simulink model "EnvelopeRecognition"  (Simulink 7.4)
settings: Solver=FixedStepDiscrete  StartTime=0.0  StopTime=10.0  RelTol=1e-3
undefined symbols (not defined in the file or in its folder): Rec, SDTV, uint
libraries: viptextngfix x3, vipconversions x3, vipsnks x2, vipmorphops x1, vipsrcs x1, dspmtrx3 x1

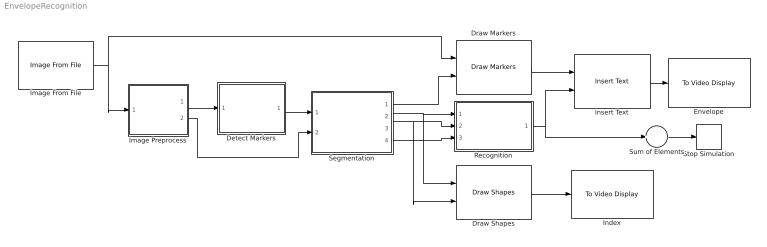
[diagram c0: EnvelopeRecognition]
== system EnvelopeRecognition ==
  Detect Markers : Subsystem
  Draw Markers : viptextngfix/Draw Markers  DialogController=vipDDGCreate  DialogControllerArgs=DataTag0  shape=X-mark  size=10  fill=on  fillClrSource=Specify via dialog  display=User-specified value  intensity=200  color=[200 255 100]  opacity=0.6  viewport=Entire image  antialiasing=off  inType=Obsolete  imagePorts=One multidimensional signal  prodOutputMode=Binary point scaling  prodOutputWordLength=32  prodOutputFracLength=14  memoryMode=Specify word length  memoryWordLength=16  memoryFracLength=15  roundingMode=Floor  overflowMode=off
  Draw Shapes : viptextngfix/Draw Shapes  DialogController=vipDDGCreate  DialogControllerArgs=DataTag1  shape=Rectangles  fill=off  fillClrSource=Specify via dialog  display=White  intensity=200  color=[0 255 0]'*ones(1, 7)  opacity=0.6  viewport=Entire image  antialiasing=off  inType=Obsolete  imagePorts=One multidimensional signal  prodOutputMode=Binary point scaling  prodOutputWordLength=32  prodOutputFracLength=14  memoryMode=Specify word length  memoryWordLength=16  memoryFracLength=15  roundingMode=Floor  overflowMode=off
  Envelope : vipsnks/To Video Display  DialogControllerArgs=DataTag2  inputType=Obsolete  imagePorts=One multidimensional signal  OutputDevice=On-screen video monitor  fullScreen=off  videoWindowX=48  videoWindowY=189  saveWindowSize=off  videoWindowWidth=1152  videoWindowHeight=757  dataOrg=Column-major  openAtMdlStart=on  isWindowOpen=off
  Image From File : vipsrcs/Image From File  Tag=vipblks_nd  DialogController=vipDDGCreate  DialogControllerArgs=DataTag3  SystemSampleTime=-1  FileName=E:\KPI\C_V_S\RGR\RELEASE\Images\DSC00377.JPG  imagePorts=One multidimensional signal  Ts=inf  ImageDataType=Inherit from input image  Signed=on  WordLength=16  sdImageDataType=uint(8)  FractionLengthMode=User-defined  FractionLength=15  OutPortLabels=R|G|B
  Image Preprocess : Subsystem
  Index : vipsnks/To Video Display  DialogControllerArgs=DataTag5  inputType=Obsolete  imagePorts=One multidimensional signal  OutputDevice=On-screen video monitor  fullScreen=off  videoWindowX=179  videoWindowY=214  saveWindowSize=off  videoWindowWidth=217  videoWindowHeight=65  dataOrg=Column-major  openAtMdlStart=on  isWindowOpen=off
  Insert Text : viptextngfix/Insert Text  DialogController=vipDDGCreate  DialogControllerArgs=DataTag6  inputType=Obsolete  theText='%s'  fontFace=Arial  dummyVar1=0  blockFontSize=48  antiAliased=on  getTextLocFrom=Specify via dialog  textLoc=[0 0]  getTextColorFrom=Specify via dialog  textColor=[0 255 0]  getTextIntensityFrom=Specify via dialog  textIntensity=0  getTextOpacityFrom=Specify via dialog  textOpacity=1.0  dummyVar2=0  dummyVar3=0  dummyVar4=0  imagePorts=One multidimensional signal  isInputTransposed=off
  Recognition : Subsystem
  Segmentation : Subsystem
  Stop Simulation : Stop
  Sum of Elements : Sum  Inputs=+  OutDataTypeMode=double  OutDataType=fixdt(1, 16)  OutScaling=2^-10  OutDataTypeStr=double
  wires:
  Image From File/1 -> Draw Markers/1, Image Preprocess/1(Image)
  Image Preprocess/1(BW) -> Detect Markers/1(BWin)
  Detect Markers/1(STATS) -> Segmentation/1(STATS)
  Segmentation/1(Pts) -> Draw Markers/2
  Image Preprocess/2(Gray) -> Segmentation/2(Image)
  Draw Shapes/1 -> Index/1
  Segmentation/2(IndexImage) -> Draw Shapes/1, Recognition/1(IndexImage)
  Segmentation/3(Rects) -> Draw Shapes/2, Recognition/2(Rects)
  Segmentation/4(Thresh) -> Recognition/3(Thresh)
  Draw Markers/1 -> Insert Text/1
  Insert Text/1 -> Envelope/1
  Recognition/1(Index) -> Insert Text/2, Sum of Elements/1
  Sum of Elements/1 -> Stop Simulation/1

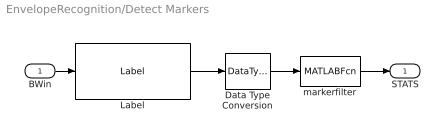
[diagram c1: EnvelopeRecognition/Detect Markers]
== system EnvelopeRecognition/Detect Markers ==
  BWin : Inport  OutDataType=fixdt(1, 16)  OutScaling=2^0
  Data Type Conversion : DataTypeConversion  OutDataTypeMode=double  OutDataType=fixdt(1, 16)  OutScaling=2^0  OutDataTypeStr=double
  Label : vipmorphops/Label  conn=8  output=Label matrix  outType=Automatic  lastLabel=maximum value of the output data type
  markerfilter : MATLABFcn  MATLABFcn=markerfilter  OutputDimensions=[7, 7]  Output1D=off
  STATS : Outport  OutDataType=fixdt(1, 16)  OutScaling=2^0
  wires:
  BWin/1 -> Label/1
  Label/1 -> Data Type Conversion/1
  markerfilter/1 -> STATS/1
  Data Type Conversion/1 -> markerfilter/1

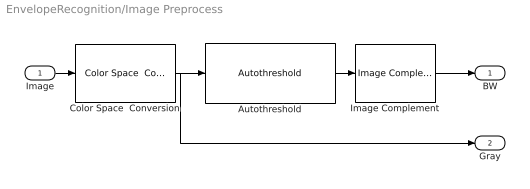
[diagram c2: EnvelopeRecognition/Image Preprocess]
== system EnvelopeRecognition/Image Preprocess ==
  Image : Inport  OutDataType=fixdt(1, 16)  OutScaling=2^0
  Autothreshold : vipconversions/Autothreshold  DialogController=vipDDGCreate  DialogControllerArgs=DataTag4  operator=>  threshOut=off  effMetricOut=off  userDefinedRange=off  umin=0  umax=255  outOfRngOpt=Warn and saturate  scaleThreshold=off  scaleFactor=1  P1Mode=Specify word length  P1WordLength=32  P1FracLength=30  P2Mode=Specify word length  P2WordLength=32  P2FracLength=22  P3Mode=Specify word length  P3WordLength=32  P3FracLength=14  P4Mode=Binary point scaling  P4WordLength=32  P4FracLength=15  Q1Mode=Specify word length  Q1WordLength=32  Q1FracLength=16  EMMode=Specify word length  EMWordLength=16  EMFracLength=14  roundingMode=Floor  overflowMode=off
  Color Space  Conversion : vipconversions/Color Space  Conversion  conversion=Obsolete  conversionActive=R'G'B' to intensity  wp_str=D65  rec=Rec. 601 (SDTV)  sys=1125/60/2:1  imagePorts=One multidimensional signal
  Image Complement : vipconversions/Image Complement
  BW : Outport  OutDataType=fixdt(1, 16)  OutScaling=2^0
  Gray : Outport  Port=2  OutDataType=fixdt(1, 16)  OutScaling=2^0
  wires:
  Image/1 -> Color Space  Conversion/1
  Color Space  Conversion/1 -> Autothreshold/1, Gray/1
  Autothreshold/1 -> Image Complement/1
  Image Complement/1 -> BW/1

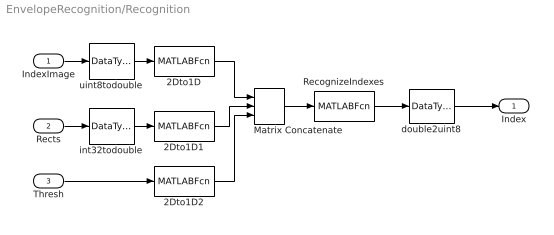
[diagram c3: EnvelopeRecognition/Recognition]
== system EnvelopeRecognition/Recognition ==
  IndexImage : Inport  OutDataType=fixdt(1, 16)  OutScaling=2^0
  Rects : Inport  Port=2  OutDataType=fixdt(1, 16)  OutScaling=2^0
  Thresh : Inport  Port=3  OutDataType=fixdt(1, 16)  OutScaling=2^0
  2Dto1D : MATLABFcn  MATLABFcn=transform2Dto1D
  2Dto1D1 : MATLABFcn  MATLABFcn=transform2Dto1D
  2Dto1D2 : MATLABFcn  MATLABFcn=transform2Dto1D
  Matrix Concatenate : Concatenate  NumInputs=3  Mode=Vector  ConcatenateDimension=2
  RecognizeIndexes : MATLABFcn  MATLABFcn=recognizeindexes  OutputDimensions=[1, 6]  Output1D=off
  double2uint8 : DataTypeConversion  OutDataTypeMode=uint8  OutDataType=fixdt(1, 16)  OutScaling=2^0  OutDataTypeStr=uint8
  int32todouble : DataTypeConversion  OutDataTypeMode=double  OutDataType=fixdt(1, 16)  OutScaling=2^0  OutDataTypeStr=double
  uint8todouble : DataTypeConversion  OutDataTypeMode=double  OutDataType=fixdt(1, 16)  OutScaling=2^0  OutDataTypeStr=double
  Index : Outport  OutDataType=fixdt(1, 16)  OutScaling=2^0
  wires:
  IndexImage/1 -> uint8todouble/1
  Rects/1 -> int32todouble/1
  Thresh/1 -> 2Dto1D2/1
  2Dto1D1/1 -> Matrix Concatenate/2
  2Dto1D/1 -> Matrix Concatenate/1
  Matrix Concatenate/1 -> RecognizeIndexes/1
  RecognizeIndexes/1 -> double2uint8/1
  double2uint8/1 -> Index/1
  uint8todouble/1 -> 2Dto1D/1
  int32todouble/1 -> 2Dto1D1/1
  2Dto1D2/1 -> Matrix Concatenate/3

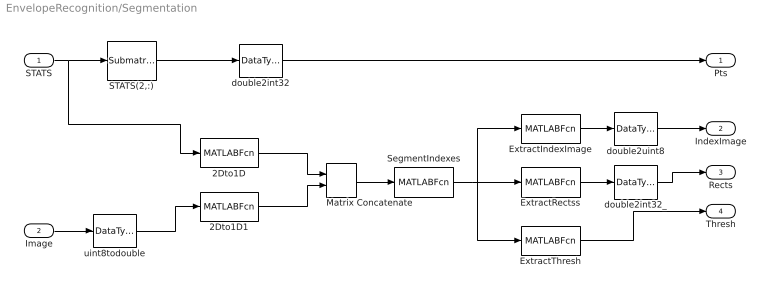
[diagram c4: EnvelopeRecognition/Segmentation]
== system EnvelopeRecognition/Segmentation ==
  STATS : Inport  OutDataType=fixdt(1, 16)  OutScaling=2^0
  Image : Inport  Port=2  OutDataType=fixdt(1, 16)  OutScaling=2^0
  2Dto1D : MATLABFcn  MATLABFcn=transform2Dto1D
  2Dto1D1 : MATLABFcn  MATLABFcn=transform2Dto1D
  ExtractIndexImage : MATLABFcn  MATLABFcn=extractindeximage  OutputDimensions=[65 217]  Output1D=off
  ExtractRectss : MATLABFcn  MATLABFcn=extractrects  OutputDimensions=[4 7]  Output1D=off
  ExtractThresh : MATLABFcn  MATLABFcn=extractthresh  OutputDimensions=[1 1]  Output1D=off
  Matrix Concatenate : Concatenate  Mode=Vector  ConcatenateDimension=2
  STATS(2,:) : dspmtrx3/Submatrix  RowSpan=Range of rows  RowStartMode=First  RowStartIndex=1  RowEndMode=Index  RowEndIndex=2  ColSpan=All columns  ColStartMode=First  ColStartIndex=1  ColEndMode=Last  ColEndIndex=1
  SegmentIndexes : MATLABFcn  MATLABFcn=segmentindexes  OutputDimensions=[65*217+4*7+1, 1]  Output1D=off
  double2int32 : DataTypeConversion  OutDataTypeMode=int32  OutDataType=fixdt(1, 16)  OutScaling=2^0  OutDataTypeStr=int32
  double2int32_ : DataTypeConversion  OutDataTypeMode=int32  OutDataType=fixdt(1, 16)  OutScaling=2^0  OutDataTypeStr=int32
  double2uint8 : DataTypeConversion  OutDataTypeMode=uint8  OutDataType=fixdt(1, 16)  OutScaling=2^0  OutDataTypeStr=uint8
  uint8todouble : DataTypeConversion  OutDataTypeMode=double  OutDataType=fixdt(1, 16)  OutScaling=2^0  OutDataTypeStr=double
  Pts : Outport  OutDataType=fixdt(1, 16)  OutScaling=2^0
  IndexImage : Outport  Port=2  OutDataType=fixdt(1, 16)  OutScaling=2^0
  Rects : Outport  Port=3  OutDataType=fixdt(1, 16)  OutScaling=2^0
  Thresh : Outport  Port=4  OutDataType=fixdt(1, 16)  OutScaling=2^0
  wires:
  STATS/1 -> STATS(2,:)/1, 2Dto1D/1
  STATS(2,:)/1 -> double2int32/1
  double2int32/1 -> Pts/1
  Image/1 -> uint8todouble/1
  2Dto1D/1 -> Matrix Concatenate/1
  2Dto1D1/1 -> Matrix Concatenate/2
  Matrix Concatenate/1 -> SegmentIndexes/1
  uint8todouble/1 -> 2Dto1D1/1
  SegmentIndexes/1 -> ExtractIndexImage/1, ExtractRectss/1, ExtractThresh/1
  ExtractIndexImage/1 -> double2uint8/1
  ExtractThresh/1 -> Thresh/1
  double2uint8/1 -> IndexImage/1
  ExtractRectss/1 -> double2int32_/1
  double2int32_/1 -> Rects/1
